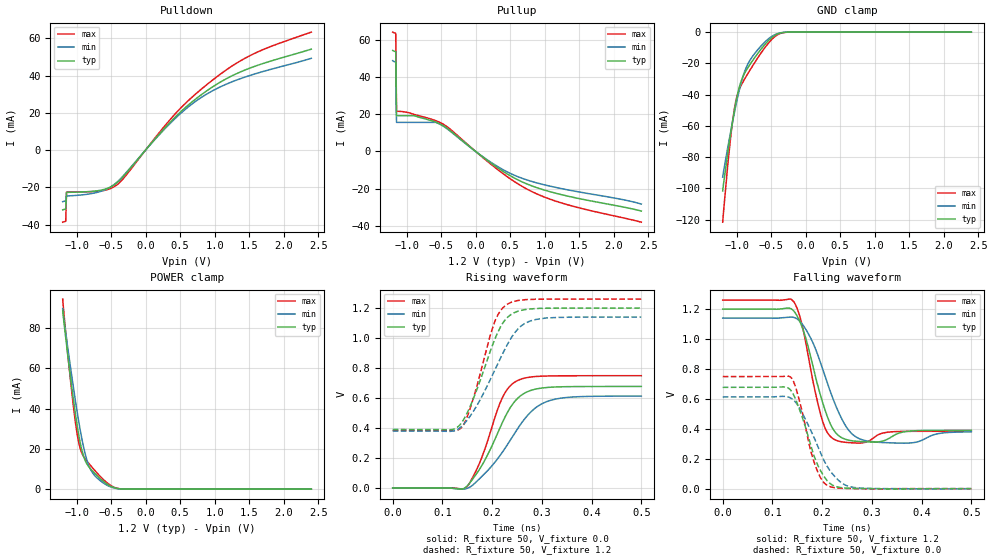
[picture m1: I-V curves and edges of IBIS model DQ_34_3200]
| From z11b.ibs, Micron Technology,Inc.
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| MODEL DQ_34_3200 (34 Ohm Data I/O with no ODT, 1600-3200Mbps)
[Model]   DQ_34_3200
Model_type   I/O
Vinl = 905.000mV
Vinh = 1015.000mV
Vmeas = 960.000mV
Vref = 1200.000mV
Cref = 0.0pF
Rref = 50.000Ohm
|   typ   min   max
|C_comp   0.780pF   0.730pF   0.830pF
C_comp_pullup   0.390pF   0.365pF   0.415pF
C_comp_pulldown   0.390pF   0.365pF   0.415pF
[Model Spec]
| Timing spec test load voltage corners
Vref   1.2000V   1.1400V   1.2600V
| Dynamic Overshoot Parameters from DDR4 Specification
|D_overshoot_ampl_h   0.40   NA   NA
|D_overshoot_ampl_l   0.40   NA   NA
|D_overshoot_area_h   0.0800n   NA   NA
|D_overshoot_area_l   0.0800n   NA   NA
[Voltage Range]   1.2000V   1.1400V   1.2600V
| Junction Temperature (Ambient temp is 35C typ, 95C min, 0C max)
[Temperature Range]   50.0   110.0   0.0
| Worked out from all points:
|   slope of the pulldown table from 0 to 0.18 V, typ, clamps not added: 23.2 ohm
|   slope of the pullup table from 0 to 0.18 V, typ, clamps not added: 35.1 ohm
|   GND clamp passes 1 mA (typ) near -0.39 V on its own axis
|   POWER clamp passes 1 mA (typ) near -0.48 V on its own axis
|   rising waveform, R_fixture 50, V_fixture 0.0: 20-80 % time 60.9ps typ, 80.1ps min, 47.6ps max; typ from 0 V to 0.677 V
|   rising waveform, R_fixture 50, V_fixture 1.2: 20-80 % time 54.5ps typ, 69.8ps min, 44.1ps max; typ from 0.39 V to 1.2 V
|   falling waveform, R_fixture 50, V_fixture 1.2: 20-80 % time 39.1ps typ, 50.6ps min, 31.9ps max; typ from 1.2 V to 0.39 V
|   falling waveform, R_fixture 50, V_fixture 0.0: 20-80 % time 41.3ps typ, 53.1ps min, 33.3ps max; typ from 0.677 V to 0 V
[Pulldown]
|   Voltage   I(typ)   I(min)   I(max)
-1.2V     -32.14mA   -27.78mA   -38.76mA
-1.156V   -31.69mA   -27.3mA    -38.27mA
-1.145V   -22.74mA   -24.67mA   -22.62mA
-687.3mV  -21.82mA   -22.61mA   -22.14mA
-523.6mV  -20.13mA   -20.2mA    -20.9mA
-414.5mV  -17.59mA   -17.26mA   -18.66mA
-283.6mV  -12.6mA    -12.21mA   -13.62mA
458.2mV   18.75mA    17.99mA    20.61mA
752.7mV   28.18mA    26.87mA    30.99mA
1.047V    35.72mA    33.3mA     39.78mA
1.571V    44.84mA    40.76mA    51.79mA
2.4V      54.19mA    49.29mA    63.35mA
[GND_clamp]
|   Voltage   I(typ)   I(min)   I(max)
-1.2V     -101.7mA   -92.86mA   -121.7mA
-1.135V   -79.96mA   -75.85mA   -88.92mA
-1.08V    -63.49mA   -62.76mA   -65.41mA
-1.036V   -51.56mA   -52.84mA   -50.64mA
-992.7mV  -41.38mA   -43.58mA   -41.02mA
-927.3mV  -30.76mA   -31.6mA    -33.57mA
-872.7mV  -25.55mA   -24.13mA   -29.29mA
-818.2mV  -21.61mA   -19.01mA   -25.29mA
-621.8mV  -9.659mA   -7.799mA   -11.96mA
-436.4mV  -1.919mA   -1.478mA   -2.611mA
-229.1mV  -17.22uA   -19.75uA   -20.83uA
2.4V      0A         0A         0A
[Pullup]
|   Voltage   I(typ)   I(min)   I(max)
-1.2V     54.34mA    48.83mA    64.24mA
-1.156V   53.69mA    48.13mA    63.56mA
-1.145V   19.23mA    15.64mA    21.64mA
-883.6mV  19.19mA    15.64mA    19.85mA
-556.4mV  15.45mA    15.34mA    16.25mA
-370.9mV  11.29mA    10.99mA    12.08mA
0V        835.2nA    819.2nA    926.2nA
338.2mV   -9.284mA   -8.558mA   -10.3mA
600mV     -15.07mA   -13.42mA   -17.15mA
883.6mV   -19.48mA   -16.91mA   -22.83mA
1.385V    -24.49mA   -21.06mA   -29.27mA
2.4V      -32.09mA   -28.34mA   -38.11mA
[Power Clamp]
|   Voltage   I(typ)   I(min)   I(max)
-1.2V     88.83mA    89.6mA     94.34mA
-1.135V   68.72mA    72.21mA    70.04mA
-1.058V   47.72mA    53.58mA    44.98mA
-1.004V   34.46mA    41.14mA    30.25mA
-960mV    25.46mA    31.98mA    21.99mA
-894.5mV  16.03mA    20.41mA    16.05mA
-807.3mV  10.5mA     10.53mA    12.15mA
-709.1mV  6.909mA    5.768mA    8.277mA
-545.5mV  2.223mA    1.735mA    2.842mA
-436.4mV  532.9uA    427.3uA    716.1uA
-294.5mV  16.21uA    18.63uA    20.69uA
2.4V      0A         0A         0A
[Ramp]
|   typ   min   max
dV/dt_r   406.22m/60.85p   367.61m/80.07p   449.27m/47.57p
dV/dt_f   486.13m/39.13p   456.28m/50.59p   526.01m/31.87p
R_load = 50
[Rising Waveform]
R_fixture = 50
V_fixture = 0.0
|   Time   V(typ)   V(min)   V(max)
0s        2.227uV    6.561uV    1.282uV
147ps     4.961mV    -5.273mV   393.9uV
158ps     46.23mV    11.58mV    52.7mV
176ps     131.7mV    66.21mV    177.1mV
221ps     439.8mV    240.3mV    605.1mV
235ps     528.3mV    311.8mV    676.4mV
253ps     603.3mV    404.5mV    719.5mV
286ps     658.3mV    531.1mV    743mV
322ps     672.8mV    588.6mV    747.6mV
500ps     677mV      612.7mV    748.8mV
[Rising Waveform]
R_fixture   = 50
V_fixture   = 1.2
V_fixture_min = 1.14
V_fixture_max = 1.26
|   Time   V(typ)   V(min)   V(max)
0s        389.8mV    380mV      383.3mV
117ps     388.7mV    377.8mV    381.9mV
139ps     437.2mV    411.6mV    405.1mV
160ps     577.2mV    500mV      574.8mV
206ps     997.1mV    790.9mV    1.116V
218ps     1.082V     874.8mV    1.188V
234ps     1.147V     976.9mV    1.232V
258ps     1.184V     1.08V      1.253V
288ps     1.197V     1.124V     1.259V
500ps     1.2V       1.14V      1.26V
[Falling Waveform]
R_fixture   = 50
V_fixture   = 1.2
V_fixture_min = 1.14
V_fixture_max = 1.26
|   Time   V(typ)   V(min)   V(max)
0s        1.2V       1.14V      1.26V
143ps     1.187V     1.144V     1.249V
159ps     1.086V     1.104V     1.103V
200ps     586mV      809.1mV    460.2mV
225ps     382.9mV    573.6mV    327.8mV
255ps     322.7mV    383.7mV    307.2mV
289ps     312.5mV    319.2mV    311.6mV
335ps     336.6mV    306.3mV    378.4mV
375ps     384.1mV    304.6mV    383mV
500ps     389.8mV    379.5mV    383.3mV
[Falling Waveform]
R_fixture = 50
V_fixture = 0.0
|   Time   V(typ)   V(min)   V(max)
0s        677.1mV    612.8mV    748.8mV
123ps     680.1mV    616.9mV    750.5mV
138ps     652.6mV    603.2mV    740.6mV
152ps     550.9mV    551.9mV    616mV
184ps     216.2mV    339.4mV    174.9mV
198ps     113.1mV    229.9mV    65.62mV
213ps     42.75mV    133.7mV    17.23mV
239ps     6.456mV    38.71mV    2.303mV
265ps     1.325mV    7.55mV     576.3uV
500ps     17.6uV     -118.9uV   6.362uV
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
